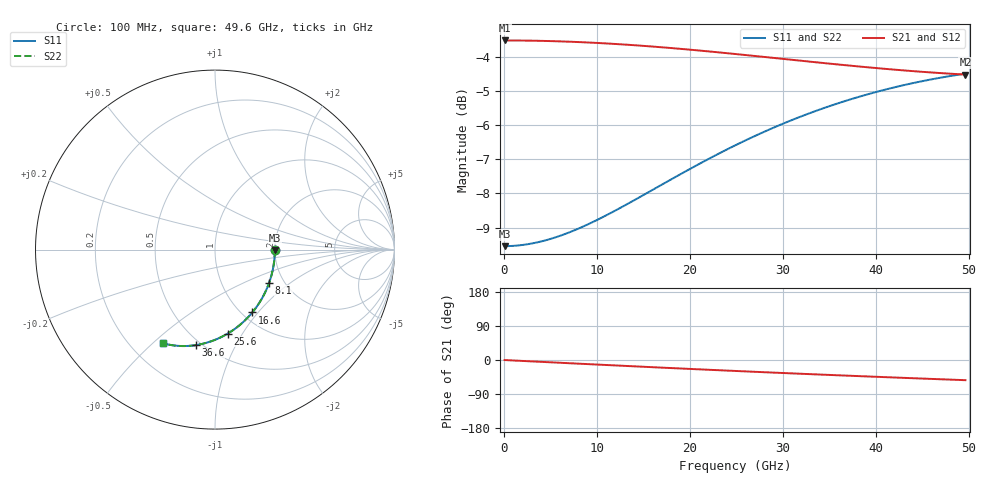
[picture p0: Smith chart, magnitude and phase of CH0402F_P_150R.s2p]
# GHz S RI R 150
! S-Parameters data
! Freq  reS11  imS11  reS21  imS21  reS12  imS12  reS22  imS22
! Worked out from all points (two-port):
!   100 points, 100 MHz to 49.6 GHz, reference 150 ohm
!   highest |S21| = -3.52 dB at 100 MHz (marker M1); lowest = -4.5 dB at 49.6 GHz (marker M2)
!   |S21| within 3 dB of the highest: start of sweep to end of sweep
!   lowest |S11| = -9.5 dB at 100 MHz (marker M3), VSWR 2.00, Z = 300 - j1.6 ohm
!   |S11| at or under -10 dB: nowhere
!   |S22| runs from -9.5 to -4.5 dB; largest |S21 - S12| = 0
!   S11 on the Smith chart (normalised r, x): 100 MHz: 2.00, -0.01; 8.1 GHz: 1.67, -0.71; 16.6 GHz: 1.11, -0.93; 25.6 GHz: 0.72, -0.86; 36.6 GHz: 0.47, -0.70; 49.6 GHz: 0.33, -0.54
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0.1  0.3333 -0.00237  0.6667 -0.0014  0.6667 -0.0014  0.3333 -0.00237
2.1  0.3311 -0.0496  0.6658 -0.0294  0.6658 -0.0294  0.3311 -0.0496
4.1  0.3249 -0.0963  0.6632 -0.0573  0.6632 -0.0573  0.3249 -0.0963
6.1  0.3148 -0.1421  0.6591 -0.0849  0.6591 -0.0849  0.3148 -0.1421
8.1  0.301 -0.1864  0.6535 -0.112  0.6535 -0.112  0.301 -0.1864
8.6  0.297 -0.1972  0.6518 -0.1187  0.6518 -0.1187  0.297 -0.1972
10.6  0.2789 -0.2392  0.6443 -0.1451  0.6443 -0.1451  0.2789 -0.2392
12.6  0.2577 -0.2789  0.6355 -0.1708  0.6355 -0.1708  0.2577 -0.2789
14.6  0.2338 -0.316  0.6254 -0.1956  0.6254 -0.1956  0.2338 -0.316
16.6  0.2076 -0.3504  0.6141 -0.2196  0.6141 -0.2196  0.2076 -0.3504
19.1  0.172 -0.3893  0.5985 -0.2481  0.5985 -0.2481  0.172 -0.3893
21.1  0.1418 -0.417  0.585 -0.2698  0.585 -0.2698  0.1418 -0.417
23.1  0.1104 -0.4417  0.5708 -0.2904  0.5708 -0.2904  0.1104 -0.4417
25.1  0.0783 -0.4632  0.5559 -0.3099  0.5559 -0.3099  0.0783 -0.4632
25.6  0.0701 -0.4682  0.5521 -0.3147  0.5521 -0.3147  0.0701 -0.4682
29.1  0.0128 -0.4975  0.5247 -0.3458  0.5247 -0.3458  0.0128 -0.4975
33.1  -0.0525 -0.5205  0.4921 -0.3777  0.4921 -0.3777  -0.0525 -0.5205
36.6  -0.108 -0.5323  0.4631 -0.4025  0.4631 -0.4025  -0.108 -0.5323
39.1  -0.1462 -0.5364  0.4423 -0.4187  0.4423 -0.4187  -0.1462 -0.5364
41.6  -0.183 -0.5373  0.4215 -0.4338  0.4215 -0.4338  -0.183 -0.5373
45.6  -0.2382 -0.5327  0.3884 -0.456  0.3884 -0.456  -0.2382 -0.5327
49.6  -0.2885 -0.5216  0.3557 -0.4761  0.3557 -0.4761  -0.2885 -0.5216
